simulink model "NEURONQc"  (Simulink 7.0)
settings: Solver=ode45  StartTime=0.0  StopTime=tstop  RelTol=1e-5
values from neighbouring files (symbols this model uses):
  I0Stim = ResSinhCorr(iRes,2)*1E-3    [ResCrV1.m]    (also in ResEnerV1.m; WaveCompIET.m = 0; WaveCompIETIf.m = 0)
  T0Stim = ResSinhCorr(iRes,1)*1E-3    [ResCrV1.m]    (also in ResEnerV1.m; WaveCompIET.m = i; WaveCompIETIf.m = i)
  TypeStim = 11    [ResCrV1.m]    (also in ResEnerV1.m; WaveCompIET.m = 5; WaveCompIETIf.m = 5)
libraries: simulink x1

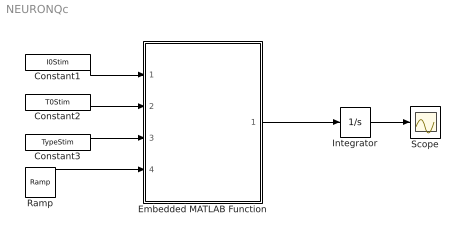
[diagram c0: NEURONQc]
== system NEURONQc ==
  Constant1 : Constant  Value=I0Stim  OutDataType=sfix(16)  OutScaling=2^0
  Constant2 : Constant  Value=T0Stim  OutDataType=sfix(16)  OutScaling=2^0
  Constant3 : Constant  Value=TypeStim  OutDataType=sfix(16)  OutScaling=2^0
  Embedded MATLAB Function : Stateflow chart
  Integrator : Integrator
  Ramp : simulink/Sources/Ramp  SystemSampleTime=-1  slope=1  start=0  X0=0
  Scope : Scope
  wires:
  Constant1/1 -> Embedded MATLAB Function/1(I0Stim)
  Constant2/1 -> Embedded MATLAB Function/2(T0Stim)
  Constant3/1 -> Embedded MATLAB Function/3(TypeStim)
  Ramp/1 -> Embedded MATLAB Function/4(temps)
  Integrator/1 -> Scope/1
  Embedded MATLAB Function/1(Istim) -> Integrator/1

== matlab function Embedded
MATLAB Function ==
function Istim = courant(I0Stim,T0Stim,TypeStim,temps)
% This block supports an embeddable subset of the MATLAB language.
% See the help menu for details. 

if temps <= T0Stim
    if TypeStim == 0
        Iout = I0Stim;
    elseif TypeStim == 1
        Iout = I0Stim*sin(pi/T0Stim*temps);
    elseif TypeStim == 2
        Iout = I0Stim*sin(pi/(2*T0Stim)*temps);
    elseif TypeStim == 3
        taum=0.07492974E-3;
        Iout = I0Stim*exp(temps/taum);
    elseif TypeStim == 4
        taum=0.07492974E-3;
        Iout = I0Stim*exp(-temps/taum);
    elseif TypeStim == 5
        Iout = I0Stim*(sin(pi/T0Stim*temps)+1/3*sin(3*pi/T0Stim*temps));
    elseif TypeStim == 6   
        taum=0.07492974E-3;
        Iout = I0Stim*sinh(temps/taum);
    elseif TypeStim == 7
        Iout = I0Stim*temps;
    elseif TypeStim == 8
        Iout = I0Stim*(T0Stim-temps);
    elseif TypeStim == 9
        Iout = I0Stim*(exp(-(5/sqrt(2))*((temps-T0Stim/2)/T0Stim)^2));
    elseif TypeStim == 10
        taum=0.2008E-3;
        Iout = I0Stim*exp(temps/taum);
    else
        taum = 4.07749143E-3;
        Iout = I0Stim*sinh(temps/taum);        
    end
else
    Iout = 0;
end
Istim = Iout;
